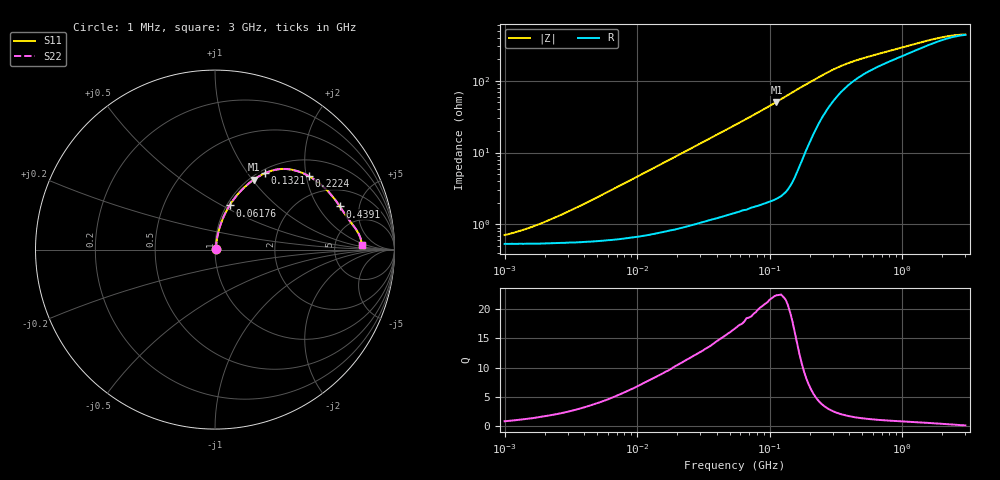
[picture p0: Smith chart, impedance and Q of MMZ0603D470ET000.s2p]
! S-Parameter Data Generated by TDK Corporation
! Copyright(C) 2025 TDK Corporation.
! All Rights Reserved.
! TDK P/N: MMZ0603D470ET000 (Chip Bead)
! Property: |Z|=47ohm at 100MHz
! Size(LxWxT): 0.6x0.3x0.3mm
! Model Type: s2p (Touchstone File Format Version 1.0)
! Frequency: DC=Yes Start=1MHz Stop=3000MHz 202points Log-sweep
! Model Generated on Feb. 6, 2025
! Terms and conditions regarding TDK Simulation Models:
! 1)This simulation model is being provided solely for informational
!  purposes. Please refer to the specifications of the products in
!  terms of detailed characteristics of such products.
! 2)In no event shall TDK Corporation of any of its subsidiaries be
!  liable for any loss or damage arising, directly or indirectly,
!  from any information contained in this simulation model, including,
!  but not limited to loss or damages arising from any inaccuracies,
!  omissions or errors in connection with such information.
! 3)Any and all copyrights on this simulation model are owned by
!  TDK Corporation.  Duplication or redistribution of this simulation
!  model without prior written permission from TDK Corporation
!  is prohibited.
! 4)This simulation model is subject to any modification or change
!  without any prior notice.
! 5)Neither TDK Corporation nor any of its subsidiaries shall make any
!  warranty, express or implied, including but not limited to the
!  correctness, implied warranties of merchantability and fitness for
!  a particular purpose with respect to this simulation models.
! 6)The use of this simulation model shall be deemed to have consented
!  to the terms and conditions hereof.
! Port Assignments:
!  1 ---@@@--- 2
! Applicable Conditions:
!  Temperature = 25 degC
!  DC Bias Current = 0 A
!  Small Signal Operation
# Hz S MA R 50
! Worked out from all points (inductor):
!   201 points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, 1 MHz to 3 GHz, reference 50 ohm
!   read as one part in series: L = 73.7 nH near 3.747 MHz
!   highest Q = 22.3 at 112.6 MHz (marker M1), where L = 71.7 nH
!   S11 on the Smith chart (normalised r, x): 1 MHz: 1.01, +0.01; 61.76 MHz: 1.03, +0.54; 132.1 MHz: 1.06, +1.21; 222.4 MHz: 1.42, +2.08; 439.1 MHz: 3.04, +3.19; 3 GHz: 9.70, +1.44
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1000000  0.007086 40.9  0.9947 -0.3  0.9947 -0.3  0.007086 40.9
1377479  0.008338 49.8  0.9946 -0.4  0.9946 -0.4  0.008338 49.8
1897447  0.01031 58.0  0.9946 -0.5  0.9946 -0.5  0.01031 58.0
3900413  0.01885 71.5  0.9942 -1.0  0.9942 -1.0  0.01885 71.5
8017732  0.03707 78.1  0.993 -2.1  0.993 -2.1  0.03707 78.1
1.461624e7  0.06597 79.7  0.9903 -3.8  0.9903 -3.8  0.06597 79.7
3.00453e7  0.1315 78.0  0.981 -7.5  0.981 -7.5  0.1315 78.0
5.477226e7  0.2317 73.2  0.959 -13.4  0.959 -13.4  0.2317 73.2
6.176144e7  0.259 71.7  0.9512 -15.0  0.9512 -15.0  0.259 71.7
8.507507e7  0.3471 66.9  0.9208 -20.3  0.9208 -20.3  0.3471 66.9
1.125904e8  0.4448 61.1  0.8759 -26.4  0.8759 -26.4  0.4448 61.1
1.321429e8  0.5085 56.8  0.8378 -30.5  0.8378 -30.5  0.5085 56.8
1.680187e8  0.5969 48.8  0.7552 -36.5  0.7552 -36.5  0.5969 48.8
2.136344e8  0.6565 39.6  0.6471 -40.3  0.6471 -40.3  0.6565 39.6
2.223601e8  0.6645 38.0  0.6277 -40.6  0.6277 -40.6  0.6645 38.0
2.609752e8  0.6906 32.0  0.5531 -41.5  0.5531 -41.5  0.6906 32.0
3.062963e8  0.7099 27.0  0.4885 -41.2  0.4885 -41.2  0.7099 27.0
4.391493e8  0.7356 19.1  0.3883 -38.3  0.3883 -38.3  0.7356 19.1
8.005644e8  0.7678 12.0  0.2954 -32.6  0.2954 -32.6  0.7678 12.0
1.931433e9  0.8115 4.9  0.2039 -20.1  0.2039 -20.1  0.8115 4.9
2.359433e9  0.8159 3.5  0.1921 -15.0  0.1921 -15.0  0.8159 3.5
3e9  0.8168 1.7  0.1852 -7.7  0.1852 -7.7  0.8168 1.7
